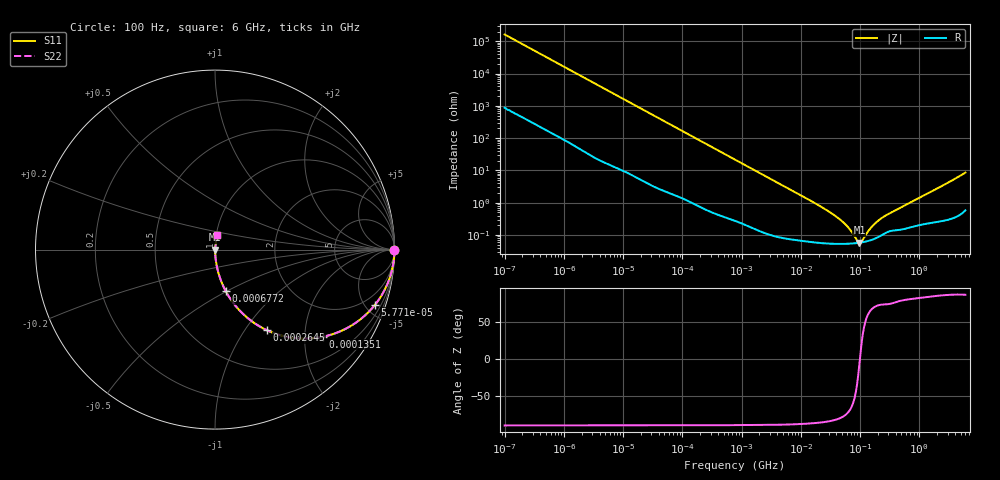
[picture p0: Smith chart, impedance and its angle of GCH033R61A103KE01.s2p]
!Murata Part Number: GCH033R61A103KE01
!These Parameters are Measured in Series Mode Connection
!Data Generated on Mar 13, 2026
!  o--ll--o
!Port1  Port2
!  o------o
!Operation Temp=25[degC], DC Bias Voltage=0[V]
!Freq. Start=100[Hz] Stop=6[GHz] 401[Steps]
# Hz S RI R 50
!Freq.(Hz) S11(Real) S11(Imag) S21(Real) S21(Imag) S12(Real) S12(Imag) S22(Real) S22(Imag)
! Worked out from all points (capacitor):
!   401 points, 100 Hz to 6 GHz, reference 50 ohm
!   read as one part in series: C = 9.78 nF near 109 Hz
!   lowest |Z| = 57.7 mohm at 97.54 MHz (marker M1)
!   series resonance near 99.48 MHz, so ESL is about 260 pH
!   S11 on the Smith chart (normalised r, x): 100 Hz: open; 57.71 kHz: 1.04, -5.76; 135.1 kHz: 1.02, -2.47; 264.5 kHz: 1.01, -1.27; 677.2 kHz: 1.01, -0.50; 6 GHz: 1.01, +0.17
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100  1 -0.000615  3.7e-06 0.000615  3.7e-06 0.000615  1 -0.000615
2008  0.9998 -0.0122  0.000212 0.0122  0.000212 0.0122  0.9998 -0.0122
12041  0.9943 -0.0725  0.00572 0.0725  0.00572 0.0725  0.9943 -0.0725
40335  0.9429 -0.2289  0.0571 0.2289  0.0571 0.2289  0.9429 -0.2289
57709  0.8906 -0.3086  0.1094 0.3086  0.1094 0.3086  0.8906 -0.3086
86348  0.786 -0.4062  0.214 0.4062  0.214 0.4062  0.786 -0.4062
135116  0.6031 -0.485  0.3969 0.485  0.3969 0.485  0.6031 -0.485
264476  0.2878 -0.4482  0.7122 0.4482  0.7122 0.4482  0.2878 -0.4482
413847  0.1436 -0.3457  0.8564 0.3457  0.8564 0.3457  0.1436 -0.3457
677235  0.0606 -0.2327  0.9394 0.2327  0.9394 0.2327  0.0606 -0.2327
774597  0.0475 -0.2065  0.9525 0.2065  0.9525 0.2065  0.0475 -0.2065
2594782  0.00535 -0.065  0.9947 0.065  0.9947 0.065  0.00535 -0.065
1.555665e7  0.000712 -0.0108  0.9993 0.0108  0.9993 0.0108  0.000712 -0.0108
4.764863e7  0.000534 -0.00279  0.9995 0.00279  0.9995 0.00279  0.000534 -0.00279
6.233367e7  0.000535 -0.00168  0.9995 0.00168  0.9995 0.00168  0.000535 -0.00168
8.918374e7  0.000561 -0.000378  0.9994 0.000378  0.9994 0.000378  0.000561 -0.000378
9.753859e7  0.000572 -6.74e-05  0.9994 6.74e-05  0.9994 6.74e-05  0.000572 -6.74e-05
1.066761e8  0.000587 0.000243  0.9994 -0.000243  0.9994 -0.000243  0.000587 0.000243
1.459435e8  0.000673 0.00135  0.9993 -0.00135  0.9993 -0.00135  0.000673 0.00135
1.825626e8  0.000787 0.0022  0.9992 -0.0022  0.9992 -0.0022  0.000787 0.0022
3.124326e8  0.00131 0.00442  0.9987 -0.00442  0.9987 -0.00442  0.00131 0.00442
6e9  0.0128 0.0836  0.9872 -0.0836  0.9872 -0.0836  0.0128 0.0836
